| Teraspeed Modeling Services.
| http://www.teraspeed.com
[IBIS Ver] 3.2
[File Name] dac34h84i.ibs
[File Rev] 3.1
[Date]   03-18-2011
[Notes]  Quality Check of this IBIS model: Model Passes IBIS Check. Model
   parses into ICX IS. Simulates with Hyperlynx.
   1. MIN TYP MAX information is based on Temperature and Voltage
   characteristics only.
   2. Package information extracted using Tektronix IConnect Software.
[Disclaimer]
| Use: Teraspeed Consulting Group LLC ("Teraspeed") has
| licensed IBIS models to specific integrated circuit
| suppliers ("IC Vendors") for use and distribustion as
| follows: Each IC Vendor may use IBIS Models, and distribute
| them to IC Vendor's custumers to use solely for developing
| printed circute board designs. Users of this model may
| modify the IBIS model to suit its specific applications but
| rights to derivative works and such modifications shall belong
| to Teraspeed. No other distribusion of these materials is
| permitted.
| DISCLAIMER OF WARRANTY: UNLESS OTHERWISE AGREED TO IN WRITING
| TERASPEED DISCLAIMS AND USER WAIVES ALL WARRANTIES, EXPRESS
| OR IMPLIED, INCLUDING WARRANTIES OF MERCHANTABILITY AND
| FITNESS FOR A PARTICULAR PURPOSE. IN NO EVENT SHALL
| TERASPEED BE LIABLE FOR ANY DIRECT OR INDIRECT DAMAGES,
| WHETHER IN CONTRACT OR TORT, INCLUDING, WITHOUT LIMITATION,
| LOST PROFITS, BUSINESS INTERRUPTION, OR LOST INFORMATION
| ARISING OUT OF THE USE OF OR THE INABILITY TO USE THE MODEL,
| EVEN IF TERASPEED HAS BEEN ADVISED OF THE POSSIBILITY OF SUCH
| DAMAGES.
[Source]
| This model file was created by Teraspeed Consulting Group LLC
| (http://www.teraspeed.com/).
[Disclaimer]
| This product is designed as an aid for customers of Texas Instruments.
| No warranties, either expressed or implied, with respect to this third
| party software (if any) or with respect to its fitness for any
| particular purpose is claimed by Texas Instruments or the author. The
| software (if any) is provided solely on an "as is" basis. The entire
| risk as to its quality and performance is with the customer
[Copyright]
| (C) Copyright 2011 Texas Instruments Incorporated. All rights reserved.
| All other rights are reserved.
[Component] DAC34H84I
[Manufacturer] TI
[Package]
| variable   typ   min   max
R_pkg  1.000E-02   1.000E-02   1.000E-02
L_pkg  1.643E-09   1.120E-09   3.139E-09
C_pkg  7.594E-13   5.322E-13   1.384E-12
[Pin] signal_name  model_name  R_pin  L_pin C_pin
A1   DAB9P   lvds_in   1.000E-02  3.139E-09  1.384E-12
A2   DAB10P   lvds_in   1.000E-02  2.908E-09  1.282E-12
A3   DAB11P   lvds_in   1.000E-02  2.700E-09  1.190E-12
A4   DAB12P   lvds_in   1.000E-02  2.521E-09  1.111E-12
A5   DAB13P   lvds_in   1.000E-02  2.378E-09  1.048E-12
A6   DAB14P   lvds_in   1.000E-02  2.278E-09  1.004E-12
A7   DAB15P   lvds_in   1.000E-02  2.226E-09  9.813E-13
A8   SYNCP   lvds_in   1.000E-02  2.226E-09  9.813E-13
A9   OSTRP   pecl_in   1.000E-02  2.278E-09  1.004E-12
A10   GND   GND   1.000E-02  1.120E-09  5.620E-13
A11   DACCLKN   pecl_in   1.000E-02  2.521E-09  1.111E-12
A12   DACCLKP   pecl_in   1.000E-02  2.700E-09  1.190E-12
A13   GND   GND   1.000E-02  1.120E-09  5.620E-13
A14   GND   GND   1.000E-02  1.120E-09  5.620E-13
B1   DAB9N   lvds_in   1.000E-02  2.908E-09  1.282E-12
B2   DAB10N   lvds_in   1.000E-02  2.656E-09  1.171E-12
B3   DAB11N   lvds_in   1.000E-02  2.427E-09  1.070E-12
B4   DAB12N   lvds_in   1.000E-02  2.226E-09  9.813E-13
B5   DAB13N   lvds_in   1.000E-02  2.063E-09  9.094E-13
B6   DAB14N   lvds_in   1.000E-02  1.947E-09  8.581E-13
B7   DAB15N   lvds_in   1.000E-02  1.886E-09  8.313E-13
B8   SYNCN   lvds_in   1.000E-02  1.886E-09  8.313E-13
B9   OSTRN   pecl_in   1.000E-02  1.947E-09  8.581E-13
B10   GND   GND   1.000E-02  1.120E-09  5.620E-13
B11   GND   GND   1.000E-02  1.120E-09  5.620E-13
B12   GND   GND   1.000E-02  1.120E-09  5.620E-13
B13   GND   GND   1.000E-02  1.120E-09  5.620E-13
B14   IOUTAP   term   1.000E-02  2.908E-09  1.282E-12
C1   DAB7N   lvds_in   1.000E-02  2.700E-09  1.190E-12
C2   DAB7P   lvds_in   1.000E-02  2.427E-09  1.070E-12
C3   DAB8N   lvds_in   1.000E-02  2.173E-09  9.579E-13
C4   DAB8P   lvds_in   1.000E-02  1.947E-09  8.581E-13
C5   GND   GND   1.000E-02  1.120E-09  5.620E-13
C6   GND   GND   1.000E-02  1.120E-09  5.620E-13
C7   GND   GND   1.000E-02  1.120E-09  5.620E-13
C8   GND   GND   1.000E-02  1.120E-09  5.620E-13
C9   GND   GND   1.000E-02  1.120E-09  5.620E-13
C10   GND   GND   1.000E-02  1.120E-09  5.620E-13
C11   PLLAVDD   POWER   1.000E-02  1.120E-09  5.620E-13
C12   CLKVDD   POWER   1.000E-02  1.120E-09  5.620E-13
C13   GND   GND   1.000E-02  1.120E-09  5.620E-13
C14   IOUTAN   term   1.000E-02  2.700E-09  1.190E-12
D1   DAB5N   lvds_in   1.000E-02  2.521E-09  1.111E-12
D2   DAB5P   lvds_in   1.000E-02  2.226E-09  9.813E-13
D3   DAB6N   lvds_in   1.000E-02  1.947E-09  8.581E-13
D4   DAB6P   lvds_in   1.000E-02  1.690E-09  7.451E-13
D5   IOVDD   POWER   1.000E-02  1.120E-09  5.620E-13
D6   IOVDD   POWER   1.000E-02  1.120E-09  5.620E-13
D7   VFUSE   POWER   1.000E-02  1.120E-09  5.620E-13
D8   GND   GND   1.000E-02  1.120E-09  5.620E-13
D9   DACVDD   POWER   1.000E-02  1.120E-09  5.620E-13
D10   AVDD   POWER   1.000E-02  1.120E-09  5.620E-13
D11   PLLAVDD   POWER   1.000E-02  1.120E-09  5.620E-13
D12   LPF   term   1.000E-02  1.947E-09  8.581E-13
D13   GND   GND   1.000E-02  1.120E-09  5.620E-13
D14   GND   GND   1.000E-02  1.120E-09  5.620E-13
E1   DAB3N   lvds_in   1.000E-02  2.378E-09  1.048E-12
E2   DAB3P   lvds_in   1.000E-02  2.063E-09  9.094E-13
E3   DAB4N   lvds_in   1.000E-02  1.758E-09  7.749E-13
E4   DAB4P   lvds_in   1.000E-02  1.469E-09  6.474E-13
E5   DIGVDD   POWER   1.000E-02  1.120E-09  5.620E-13
E6   DIGVDD   POWER   1.000E-02  1.120E-09  5.620E-13
E7   DIGVDD   POWER   1.000E-02  1.120E-09  5.620E-13
E8   GND   GND   1.000E-02  1.120E-09  5.620E-13
E9   DACVDD   POWER   1.000E-02  1.120E-09  5.620E-13
E10   DACVDD   POWER   1.000E-02  1.120E-09  5.620E-13
 E11  AVDD   POWER   1.000E-02  1.120E-09  5.620E-13
E12   GND   GND   1.000E-02  1.120E-09  5.620E-13
E13   GND   GND   1.000E-02  1.120E-09  5.620E-13
E14   IOUTBP   term   1.000E-02  2.378E-09  1.048E-12
F1   DAB1N   lvds_in   1.000E-02  2.278E-09  1.004E-12
F2   DAB1P   lvds_in   1.000E-02  1.947E-09  8.581E-13
F3   DAB2N   lvds_in   1.000E-02  1.620E-09  7.140E-13
F4   DAB2P   lvds_in   1.000E-02  1.300E-09  5.732E-13
F5   DIGVDD   POWER   1.000E-02  1.120E-09  5.620E-13
F6   GND   GND   1.000E-02  1.120E-09  5.620E-13
F7   GND   GND   1.000E-02  1.120E-09  5.620E-13
F8   GND   GND   1.000E-02  1.120E-09  5.620E-13
F9   GND   GND   1.000E-02  1.120E-09  5.620E-13
F10   DACVDD   POWER   1.000E-02  1.120E-09  5.620E-13
 F11  AVDD   POWER   1.000E-02  1.120E-09  5.620E-13
F12   GND   GND   1.000E-02  1.120E-09  5.620E-13
F13   GND   GND   1.000E-02  1.120E-09  5.620E-13
F14   IOUTBN   term   1.000E-02  2.278E-09  1.004E-12
G1   DATACLKN   lvds_in   1.000E-02  2.226E-09  9.813E-13
G2   DATACLKP   lvds_in   1.000E-02  1.886E-09  8.313E-13
G3   DAB0N   lvds_in   1.000E-02  1.546E-09  6.815E-13
G4   DAB0P   lvds_in   1.000E-02  1.207E-09  5.322E-13
G5   IOVDD   POWER   1.000E-02  1.120E-09  5.620E-13
G6   GND   GND   1.000E-02  1.120E-09  5.620E-13
G7   GND   GND   1.000E-02  1.120E-09  5.620E-13
G8   GND   GND   1.000E-02  1.120E-09  5.620E-13
G9   GND   GND   1.000E-02  1.120E-09  5.620E-13
G10   DACVDD   POWER   1.000E-02  1.120E-09  5.620E-13
 G11  AVDD   POWER   1.000E-02  1.120E-09  5.620E-13
G12   EXTIO   term   1.000E-02  1.546E-09  6.815E-13
G13   GND   GND   1.000E-02  1.120E-09  5.620E-13
G14   GND   GND   1.000E-02  1.120E-09  5.620E-13
H1   ISTRN/PARABN  lvds_in   1.000E-02  2.226E-09  9.813E-13
H2   ISTRP/PARABP  lvds_in   1.000E-02  1.886E-09  8.313E-13
H3   DCD15N   lvds_in   1.000E-02  1.546E-09  6.815E-13
H4   DCD15P   lvds_in   1.000E-02  1.207E-09  5.322E-13
H5   IOVDD   POWER   1.000E-02  1.120E-09  5.620E-13
H6   GND   GND   1.000E-02  1.120E-09  5.620E-13
H7   GND   GND   1.000E-02  1.120E-09  5.620E-13
H8   GND   GND   1.000E-02  1.120E-09  5.620E-13
H9   GND   GND   1.000E-02  1.120E-09  5.620E-13
H10   DACVDD   POWER   1.000E-02  1.120E-09  5.620E-13
H11   AVDD   POWER   1.000E-02  1.120E-09  5.620E-13
H12   BIASJ   term   1.000E-02  1.546E-09  6.815E-13
H13   GND   GND   1.000E-02  1.120E-09  5.620E-13
H14   GND   GND   1.000E-02  1.120E-09  5.620E-13
J1   DCD13N   lvds_in   1.000E-02  2.278E-09  1.004E-12
J2   DCD13P   lvds_in   1.000E-02  1.947E-09  8.581E-13
J3   DCD14N   lvds_in   1.000E-02  1.620E-09  7.140E-13
J4   DCD14P   lvds_in   1.000E-02  1.300E-09  5.732E-13
J5   DIGVDD   POWER   1.000E-02  1.120E-09  5.620E-13
J6   GND   GND   1.000E-02  1.120E-09  5.620E-13
J7   GND   GND   1.000E-02  1.120E-09  5.620E-13
J8   GND   GND   1.000E-02  1.120E-09  5.620E-13
J9   GND   GND   1.000E-02  1.120E-09  5.620E-13
J10   DACVDD   POWER   1.000E-02  1.120E-09  5.620E-13
 J11  AVDD   POWER   1.000E-02  1.120E-09  5.620E-13
J12   GND   GND   1.000E-02  1.120E-09  5.620E-13
J13   GND   GND   1.000E-02  1.120E-09  5.620E-13
J14   IOUTCP   term   1.000E-02  2.278E-09  1.004E-12
K1   DCD11N   lvds_in   1.000E-02  2.378E-09  1.048E-12
K2   DCD11P   lvds_in   1.000E-02  2.063E-09  9.094E-13
K3   DCD12N   lvds_in   1.000E-02  1.758E-09  7.749E-13
K4   DCD12P   lvds_in   1.000E-02  1.469E-09  6.474E-13
K5   DIGVDD   POWER   1.000E-02  1.120E-09  5.620E-13
K6   DIGVDD   POWER   1.000E-02  1.120E-09  5.620E-13
K7   DIGVDD   POWER   1.000E-02  1.120E-09  5.620E-13
K8   GND   GND   1.000E-02  1.120E-09  5.620E-13
K9   DACVDD   POWER   1.000E-02  1.120E-09  5.620E-13
K10   DACVDD   POWER   1.000E-02  1.120E-09  5.620E-13
K11  AVDD   POWER   1.000E-02  1.120E-09  5.620E-13
K12   CLKVDD   POWER   1.000E-02  1.120E-09  5.620E-13
K13   GND   GND   1.000E-02  1.120E-09  5.620E-13
K14   IOUTCN   term   1.000E-02  2.378E-09  1.048E-12
L1   DCD9N   lvds_in   1.000E-02  2.521E-09  1.111E-12
L2   DCD9P   lvds_in   1.000E-02  2.226E-09  9.813E-13
L3   DCD10N   lvds_in   1.000E-02  1.947E-09  8.581E-13
L4   DCD10P   lvds_in   1.000E-02  1.690E-09  7.451E-13
L5   IOVDD   POWER   1.000E-02  1.120E-09  5.620E-13
L6   IOVDD   POWER   1.000E-02  1.120E-09  5.620E-13
L7   VFUSE   POWER   1.000E-02  1.120E-09  5.620E-13
L8   GND   GND   1.000E-02  1.120E-09  5.620E-13
L9   DACVDD   POWER   1.000E-02  1.120E-09  5.620E-13
L10   AVDD   POWER   1.000E-02  1.120E-09  5.620E-13
L11   TESTMODE   NC   1.000E-02  1.120E-09  5.620E-13
L12   IOVDD2   POWER   1.000E-02  1.120E-09  5.620E-13
L13   GND   GND   1.000E-02  1.120E-09  5.620E-13
L14   GND   GND   1.000E-02  1.120E-09  5.620E-13
M1   DCD7N   lvds_in   1.000E-02  2.700E-09  1.190E-12
M2   DCD7P   lvds_in   1.000E-02  2.427E-09  1.070E-12
M3   DCD8N   lvds_in   1.000E-02  2.173E-09  9.579E-13
M4   DCD8P   lvds_in   1.000E-02  1.947E-09  8.581E-13
M5   GND   GND   1.000E-02  1.120E-09  5.620E-13
M6   GND   GND   1.000E-02  1.120E-09  5.620E-13
M7   GND   GND   1.000E-02  1.120E-09  5.620E-13
M8   GND   GND   1.000E-02  1.120E-09  5.620E-13
M9   GND   GND   1.000E-02  1.120E-09  5.620E-13
M10   GND   GND   1.000E-02  1.120E-09  5.620E-13
M11   GND   GND   1.000E-02  1.120E-09  5.620E-13
M12   GND   GND   1.000E-02  1.120E-09  5.620E-13
M13   GND   GND   1.000E-02  1.120E-09  5.620E-13
M14   IOUTDP   term   1.000E-02  2.700E-09  1.190E-12
N1   DCD6P   lvds_in   1.000E-02  2.908E-09  1.282E-12
N2   DCD5P   lvds_in   1.000E-02  2.656E-09  1.171E-12
N3   DCD4P   lvds_in   1.000E-02  2.427E-09  1.070E-12
N4   DCD3P   lvds_in   1.000E-02  2.226E-09  9.813E-13
N5   DCD2P   lvds_in   1.000E-02  2.063E-09  9.094E-13
N6   DCD1P   lvds_in   1.000E-02  1.947E-09  8.581E-13
N7   DCD0P   lvds_in   1.000E-02  1.886E-09  8.313E-13
N8   PARITYCDP   lvds_in   1.000E-02  1.886E-09  8.313E-13
N9   TXENB   in_pd   1.000E-02  1.947E-09  8.581E-13
N10   RESETB   in_pu   1.000E-02  2.063E-09  9.094E-13
N11   SLEEP   in_pd   1.000E-02  2.226E-09  9.813E-13
N12   ALARM   alarm_tri 1.000E-02  2.427E-09  1.070E-12
N13   GND   GND   1.000E-02  1.120E-09  5.620E-13
N14   IOUTDN   term   1.000E-02  2.908E-09  1.282E-12
P1   DCD6N   lvds_in   1.000E-02  3.139E-09  1.384E-12
P2   DCD5N   lvds_in   1.000E-02  2.908E-09  1.282E-12
P3   DCD4N   lvds_in   1.000E-02  2.700E-09  1.190E-12
P4   DCD3N   lvds_in   1.000E-02  2.521E-09  1.111E-12
P5   DCD2N   lvds_in   1.000E-02  2.378E-09  1.048E-12
P6   DCD1N   lvds_in   1.000E-02  2.278E-09  1.004E-12
P7   DCD0N   lvds_in   1.000E-02  2.226E-09  9.813E-13
P8   PARITYCDN   lvds_in   1.000E-02  2.226E-09  9.813E-13
P9   SCLK   in_sclk   1.000E-02  2.278E-09  1.004E-12
P10   SDENB   in_pu   1.000E-02  2.378E-09  1.048E-12
P11   SDIO   spi_io   1.000E-02  2.521E-09  1.111E-12
P12   SDO   spi_tri   1.000E-02  2.700E-09  1.190E-12
P13   GND   GND   1.000E-02  1.120E-09  5.620E-13
P14   GND   GND   1.000E-02  1.120E-09  5.620E-13
[Diff Pin] inv_pin vdiff tdelay_typ tdelay_min tdelay_max
A9  B9  400mV   NA  NA  NA
A12 A11 400mV   NA  NA  NA
G4  G3  150mV   NA  NA  NA
A2  B2  150mV   NA  NA  NA
A3  B3  150mV   NA  NA  NA
A4  B4  150mV   NA  NA  NA
A5  B5  150mV   NA  NA  NA
A6  B6  150mV   NA  NA  NA
A7  B7  150mV   NA  NA  NA
F2  F1  150mV   NA  NA  NA
F4  F3  150mV   NA  NA  NA
E2  E1  150mV   NA  NA  NA
E4  E3  150mV   NA  NA  NA
D2  D1  150mV   NA  NA  NA
D4  D3  150mV   NA  NA  NA
C2  C1  150mV   NA  NA  NA
C4  C3  150mV   NA  NA  NA
A1  B1  150mV   NA  NA  NA
G2  G1  150mV   NA  NA  NA
N7  P7  150mV   NA  NA  NA
L4  L3  150mV   NA  NA  NA
K2  K1  150mV   NA  NA  NA
K4  K3  150mV   NA  NA  NA
J2  J1  150mV   NA  NA  NA
J4  J3  150mV   NA  NA  NA
H4  H3  150mV   NA  NA  NA
N6  P6  150mV   NA  NA  NA
N5  P5  150mV   NA  NA  NA
N4  P4  150mV   NA  NA  NA
N3  P3  150mV   NA  NA  NA
N2  P2  150mV   NA  NA  NA
N1  P1  150mV   NA  NA  NA
M2  M1  150mV   NA  NA  NA
M4  M3  150mV   NA  NA  NA
L2  L1  150mV   NA  NA  NA
H2  H1  150mV   NA  NA  NA
N8  P8  150mV   NA  NA  NA
A8  B8  150mV   NA  NA  NA
[Series Pin Mapping] pin_2 model_name function_table_group
G4  G3  110ohm
A2  B2  110ohm
A3  B3  110ohm
A4  B4  110ohm
A5  B5  110ohm
A6  B6  110ohm
A7  B7  110ohm
F2  F1  110ohm
F4  F3  110ohm
E2  E1  110ohm
E4  E3  110ohm
D2  D1  110ohm
D4  D3  110ohm
C2  C1  110ohm
C4  C3  110ohm
A1  B1  110ohm
G2  G1  110ohm
N7  P7  110ohm
L4  L3  110ohm
K2  K1  110ohm
K4  K3  110ohm
J2  J1  110ohm
J4  J3  110ohm
H4  H3  110ohm
N6  P6  110ohm
N5  P5  110ohm
N4  P4  110ohm
N3  P3  110ohm
N2  P2  110ohm
N1  P1  110ohm
M2  M1  110ohm
M4  M3  110ohm
L2  L1  110ohm
H2  H1  110ohm
N8  P8  110ohm
A8  B8  110ohm
[Model selector] in_pd
pd_1.8v  input w/int pulldown,vddio2=1.8v
pd_2.5v  input w/int pulldown,vddio2=2.5v
pd_3.3v  input w/int pulldown,vddio2=3.3v
[Model selector] in_pu
pu_1.8v  input w/int pullup,vddio2=1.8v
pu_2.5v  input w/int pullup,vddio2=2.5v
pu_3.3v  input w/int pullup,vddio2=3.3v
[Model selector] in_sclk
sclk_1.8v  sclk input,vddio2=1.8v
sclk_2.5v  sclk input,vddio2=2.5v
sclk_3.3v  sclk input,vddio2=3.3v
[Model selector] spi_tri
sdo_1.8v  3-state spi output,vddio2=1.8v
sdo_2.5v  3-state spi output,vddio2=2.5v
sdo_3.3v  3-state spi output,vddio2=3.3v
[Model selector] spi_io
sdio_1.8v  bidir spi output,vddio2=1.8v
sdio_2.5v  bidir spi output,vddio2=2.5v
sdio_3.3v  bidir spi output,vddio2=3.3v
[Model selector] alarm_tri
alarm_1.8v  3-state alarm output,vddio2=1.8v
alarm_2.5v  3-state alarm output,vddio2=2.5v
alarm_3.3v  3-state alarm output,vddio2=3.3v
[Model]  110ohm
Model_type Series
C_comp   0   0   0
[Voltage Range]  3.300   3.00   3.60
[Temperature Range] 25   125   -40
[R series]   110   85   135
[Model]  term
Model_type Terminator
C_comp   0   0   0
[Voltage Range]  3.30  3.00  3.60
[Temperature Range] 25   125   -40
| Models and submodels in the file (22): lvds_in (Input), pd_1.8v (Input), pd_2.5v (Input), pd_3.3v (Input), pecl_in (Input), pu_1.8v (Input), pu_2.5v (Input), pu_3.3v (Input), sclk_1.8v (Input), sclk_2.5v (Input), sclk_3.3v (Input), alarm_1.8v (3-state), alarm_2.5v (3-state), alarm_3.3v (3-state), sdio_1.8v (I/O), sdio_2.5v (I/O), sdio_3.3v (I/O), sdo_1.8v (3-state), sdo_2.5v (3-state), sdo_3.3v (3-state), 110ohm (Series), term (Terminator)
